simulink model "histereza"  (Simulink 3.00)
settings: Solver=ode45  StartTime=0.0  StopTime=10.0  RelTol=1e-3

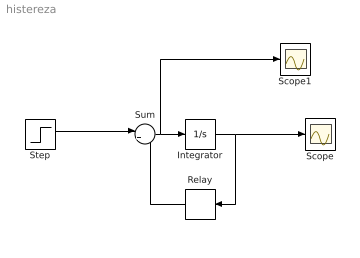
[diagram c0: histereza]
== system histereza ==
  Integrator : Integrator  ExternalReset=none  InitialConditionSource=internal  InitialCondition=0  LimitOutput=off  UpperSaturationLimit=inf  LowerSaturationLimit=-inf  ShowSaturationPort=off  ShowStatePort=off  AbsoluteTolerance=auto
  Relay : Relay  Orientation=left  OnSwitchValue=1  OffSwitchValue=-1  OnOutputValue=-1  OffOutputValue=1
  Scope : Scope
  Scope1 : Scope
  Step : Step  Time=0  Before=0  After=0.5  SampleTime=0
  Sum : Sum  Inputs=|++  SaturateOnIntegerOverflow=on
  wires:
  Step/1 -> Sum/1
  Sum/1 -> Integrator/1, Scope1/1
  Integrator/1 -> Relay/1, Scope/1
  Relay/1 -> Sum/2
